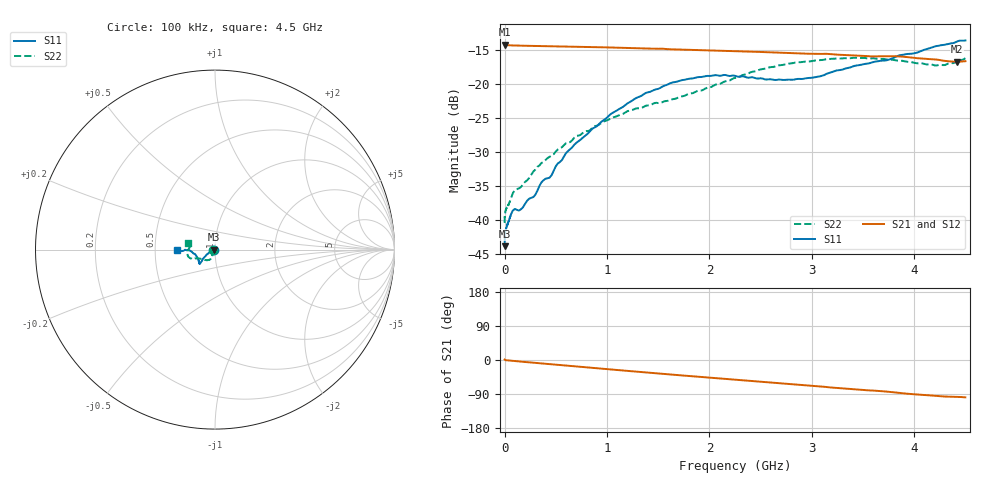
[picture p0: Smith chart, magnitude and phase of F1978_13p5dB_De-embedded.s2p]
! Integrated Device Technology
! Corporate Headquarters
! 6024 Silver Creek Valley Road
! San Jose, CA 95138  USA
! Phone:  1-408-284-8200
! Toll Free:  1-800-223-1366
! Webpage:  http://www.idt.com/
! Timing and RF Division
! 515 Groton Road, Suite 102
! Westford, MA 01886-6024
! Device:  F1978
! Description: 6-bit, 75 ohm, 0.5 dB Digital Step Attenuator
! Frequency:  5.0 MHz -  3.00 GHz
! Package:  4x4 mm QFN Plastic Package: 20 pin
! Ports:  2 RF, 11 DC
!  Pin  1  = D5 (16 dB)
!  Pin  2  = RF1  =  Port 1
!  Pin  3  = Serial Data In (DATA)
!  Pin  4  = Serial Clock (CLK)
!  Pin  5  = Serial Latch Enable (LE)
!  Pin  6  = VDD
!  Pin  7  = NC
!  Pin  8  = NC
!  Pin  9  = NC
!  Pin 10  = GND
!  Pin 11  = GND
!  Pin 12  = NC
!  Pin 13  = VMODE
!  Pin 14  = RF2  =  Port 2
!  Pin 15  = D4 (8 dB)
!  Pin 16  = D3 (4 dB)
!  Pin 17  = D2 (2 dB)
!  Pin 18  = NC
!  Pin 19  = D1 (1 dB)
!  Pin 20  = D0 (0.5 dB)
! State:  27
! Atten State:  13.5 dB
! Voltage:  +3.30 Volts
! Current:  0.561 mA
! Data:  The device was measured on a F1975 evaluation board which has
!  individual transmission lines to the RF pins.  Data was collected
!  using a calibrated network analyzer.  The evaluation board was
!  de-embedded using Automatic Fixture Removal (AFR).
!  The reference plane is the edge of the package pin.
! Misc:
!  Action Tracker AT0416
! Date Measured:  2018-02-08
! Date:  2018-03-26  MJV
! Note:
!  Integrated Device Technology supplies this data as a sample of measured
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# GHz S dB R 75
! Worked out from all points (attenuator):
!   291 points, 100 kHz to 4.5 GHz, reference 75 ohm
!   highest |S21| = -14.17 dB at 100 kHz (marker M1); lowest = -16.7 dB at 4.42 GHz (marker M2)
!   lowest |S11| = -43.8 dB at 100 kHz (marker M3), VSWR 1.01, Z = 74 + j0.0099 ohm
!   |S11| at or under -10 dB: start of sweep to end of sweep
!   |S22| runs from -40.4 to -16.1 dB; largest |S21 - S12| = 0.00016
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0.0001  -43.83 179.4  -14.17 1.2  -14.17 1.2  -40.40 -178.1
0.0006  -42.93 -176.9  -14.19 1.1  -14.18 1.1  -39.83 -176.5
0.002  -42.36 -175.4  -14.21 0.8  -14.20 0.8  -39.38 -175.1
0.011  -41.36 -172.9  -14.24 -0.5  -14.24 -0.5  -38.50 -171.4
0.08  -38.59 -165.1  -14.29 -2.3  -14.29 -2.3  -36.04 -156.6
0.16  -38.39 -160.6  -14.33 -4.2  -14.33 -4.2  -35.13 -138.5
0.28  -36.61 -158.9  -14.36 -7.1  -14.36 -7.1  -32.86 -127.8
0.36  -34.44 -159.8  -14.39 -9.0  -14.39 -9.0  -31.59 -120.5
0.44  -33.73 -157.4  -14.41 -10.9  -14.41 -10.9  -30.68 -115.5
0.6  -30.13 -156.6  -14.46 -14.7  -14.46 -14.7  -28.67 -114.0
0.76  -27.92 -151.4  -14.50 -18.4  -14.50 -18.4  -27.21 -113.7
1.04  -24.35 -147.0  -14.59 -25.0  -14.59 -25.0  -25.01 -114.9
1.38  -21.27 -142.0  -14.74 -32.8  -14.74 -32.8  -23.16 -122.7
1.52  -20.55 -139.2  -14.77 -35.9  -14.76 -35.9  -22.74 -126.6
1.88  -18.98 -137.1  -14.97 -43.9  -14.97 -43.9  -21.02 -141.9
2.26  -18.80 -139.6  -15.12 -52.3  -15.12 -52.3  -19.05 -153.6
2.64  -19.37 -150.4  -15.32 -60.6  -15.32 -60.6  -17.40 -158.1
3.02  -19.00 -165.5  -15.52 -68.6  -15.52 -68.6  -16.55 -162.2
3.76  -16.34 -178.6  -15.86 -84.1  -15.85 -84.1  -16.38 -176.8
4.22  -14.38 -177.8  -16.37 -94.9  -16.37 -94.9  -17.24 170.4
4.42  -13.70 -177.1  -16.70 -97.4  -16.69 -97.4  -16.59 168.1
4.5  -13.56 -179.0  -16.61 -98.6  -16.61 -98.6  -16.17 166.9
